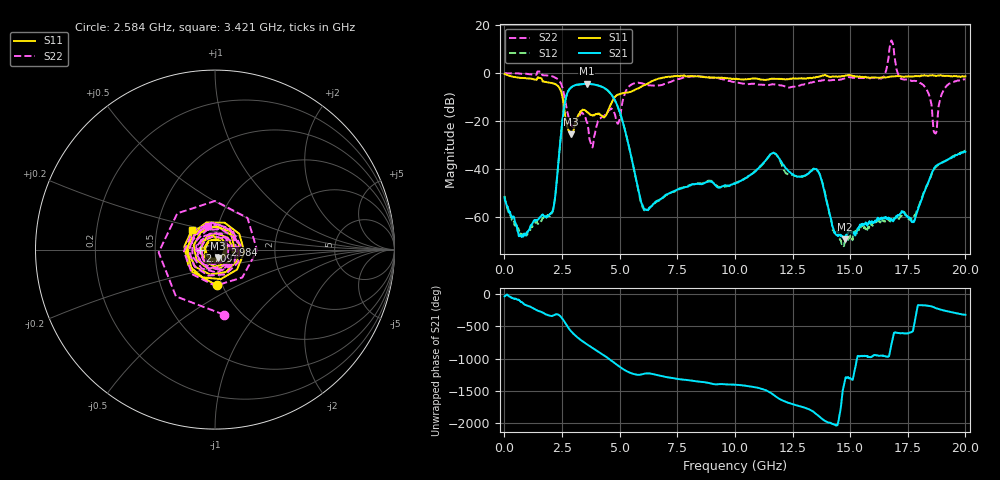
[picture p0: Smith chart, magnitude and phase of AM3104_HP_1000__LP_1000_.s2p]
!Created with skrf (http://scikit-rf.org).
# Hz S RI R 50.0
!freq ReS11 ImS11 ReS21 ImS21 ReS12 ImS12 ReS22 ImS22
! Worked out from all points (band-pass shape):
!   1601 points, 10 MHz to 20 GHz, reference 50 ohm
!   highest |S21| = -4.47 dB at 3.571 GHz (marker M1); lowest = -69.5 dB at 14.77 GHz (marker M2)
!   |S21| within 3 dB of the highest: 2.772 GHz to 4.513 GHz (1.74 GHz wide, 47.8 % of centre)
!   lowest |S11| = -25.6 dB at 2.896 GHz (marker M3), VSWR 1.11, Z = 51.4 - j5.12 ohm
!   |S11| at or under -10 dB: 2.52 GHz to 4.792 GHz (2.272 GHz wide, 62.1 % of centre)
!   |S22| runs from -31.1 to 13.7 dB; largest |S21 - S12| = 0.043
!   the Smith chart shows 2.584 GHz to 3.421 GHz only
!   S11 on the Smith chart (normalised r, x): 2.584 GHz: 0.94, -0.39; 2.709 GHz: 0.85, -0.01; 2.984 GHz: 1.11, +0.06; 3.421 GHz: 0.75, +0.17
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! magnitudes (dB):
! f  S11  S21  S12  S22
! 10 MHz  -0.4  -52.0  -51.3  -0.1
! 722.1 MHz  -2.0  -68.0  -67.5  -0.3
! 2.021 GHz  -4.1  -58.6  -58.8  -1.2
! 2.584 GHz  -14.1  -14.9  -14.9  -8.7
! 2.709 GHz  -21.6  -9.0  -8.9  -15.2
! 2.896 GHz  -25.6  -6.0  -6.1  -22.1
! 2.984 GHz  -24.6  -5.4  -5.4  -22.2
! 3.346 GHz  -15.7  -4.6  -4.7  -16.6
! 3.421 GHz  -15.4  -4.6  -4.6  -17.2
! 3.571 GHz  -16.1  -4.5  -4.6  -20.4
! 4.845 GHz  -9.5  -12.4  -12.4  -19.6
! 6.019 GHz  -5.2  -55.9  -56.5  -4.4
! 6.682 GHz  -2.3  -53.4  -53.5  -5.2
! 10.01 GHz  -2.5  -46.3  -46.1  -3.9
! 11.64 GHz  -2.4  -33.5  -33.4  -4.6
! 13.34 GHz  -2.1  -40.8  -40.7  -3.9
! 14.77 GHz  -1.1  -69.5  -71.1  -2.2
! 16.68 GHz  -1.6  -61.0  -61.6  7.2
! 17.75 GHz  -1.3  -61.7  -60.4  -3.2
! 18.68 GHz  -1.0  -39.3  -39.7  -25.1
! 19.09 GHz  -1.2  -37.0  -36.9  -6.5
! 20 GHz  -1.4  -33.0  -32.5  -2.6
